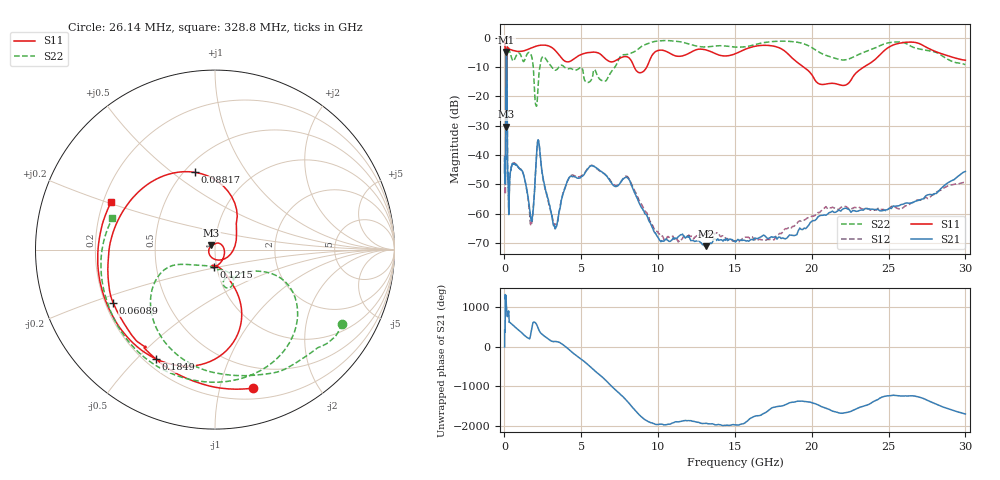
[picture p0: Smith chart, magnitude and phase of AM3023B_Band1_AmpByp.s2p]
# Hz S DB R 50.0
!freq dBS11 angS11 dBS21 angS21 dBS12 angS12 dBS22 angS22
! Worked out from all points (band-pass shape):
!   1601 points, 10 MHz to 30 GHz, reference 50 ohm
!   highest |S21| = -4.88 dB at 120.9 MHz (marker M1); lowest = -71.1 dB at 13.14 GHz (marker M2)
!   |S21| within 3 dB of the highest: 96.21 MHz to 160.7 MHz (64.47 MHz wide, 50.2 % of centre)
!   lowest |S11| = -30.4 dB at 103 MHz (marker M3), VSWR 1.06, Z = 48 + j2.2 ohm
!   |S11| at or under -10 dB: 91.17 MHz to 158.8 MHz (67.65 MHz wide, 54.1 % of centre); 8.446 GHz to 9.261 GHz (815.4 MHz wide, 9.21 % of centre); 19.48 GHz to 23.38 GHz (3.906 GHz wide, 18.2 % of centre)
!   |S22| runs from -23.3 to -0.9 dB; largest |S21 - S12| = 0.013
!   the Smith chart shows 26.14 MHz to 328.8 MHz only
!   S11 on the Smith chart (normalised r, x): 26.14 MHz: 0.29, -1.27; 60.89 MHz: 0.23, -0.23; 88.17 MHz: 0.57, +0.61; 121.5 MHz: 0.97, -0.19; 184.9 MHz: 0.24, -0.57; 328.8 MHz: 0.23, +0.21
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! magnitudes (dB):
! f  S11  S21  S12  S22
! 10 MHz  -1.0  -41.2  -40.6  -1.3
! 26.14 MHz  -1.9  -42.0  -41.6  -1.7
! 38.04 MHz  -3.0  -42.7  -42.3  -1.8
! 60.89 MHz  -3.9  -47.9  -50.0  -2.8
! 78.98 MHz  -5.1  -40.0  -40.2  -4.4
! 88.17 MHz  -7.0  -19.6  -19.6  -9.0
! 103 MHz  -30.4  -5.7  -5.6  -19.1
! 120.9 MHz  -20.5  -4.9  -4.8  -12.9
! 121.5 MHz  -20.4  -4.9  -4.8  -12.9
! 144.7 MHz  -16.5  -5.2  -5.1  -14.4
! 184.9 MHz  -3.2  -28.9  -28.9  -3.0
! 274.6 MHz  -3.8  -59.5  -58.8  -3.6
! 328.8 MHz  -3.9  -49.5  -50.3  -4.5
! 547.7 MHz  -4.4  -42.9  -43.0  -7.9
! 1.731 GHz  -3.5  -62.3  -64.1  -5.8
! 2.084 GHz  -2.8  -40.2  -40.1  -23.3
! 2.445 GHz  -2.5  -45.7  -46.2  -6.7
! 3.285 GHz  -4.2  -65.2  -63.6  -11.1
! 4.283 GHz  -8.0  -47.3  -47.3  -10.5
! 7.926 GHz  -6.4  -47.6  -47.2  -5.7
! 13.14 GHz  -4.2  -71.1  -67.1  -3.1
! 30 GHz  -7.7  -45.6  -49.3  -9.2
